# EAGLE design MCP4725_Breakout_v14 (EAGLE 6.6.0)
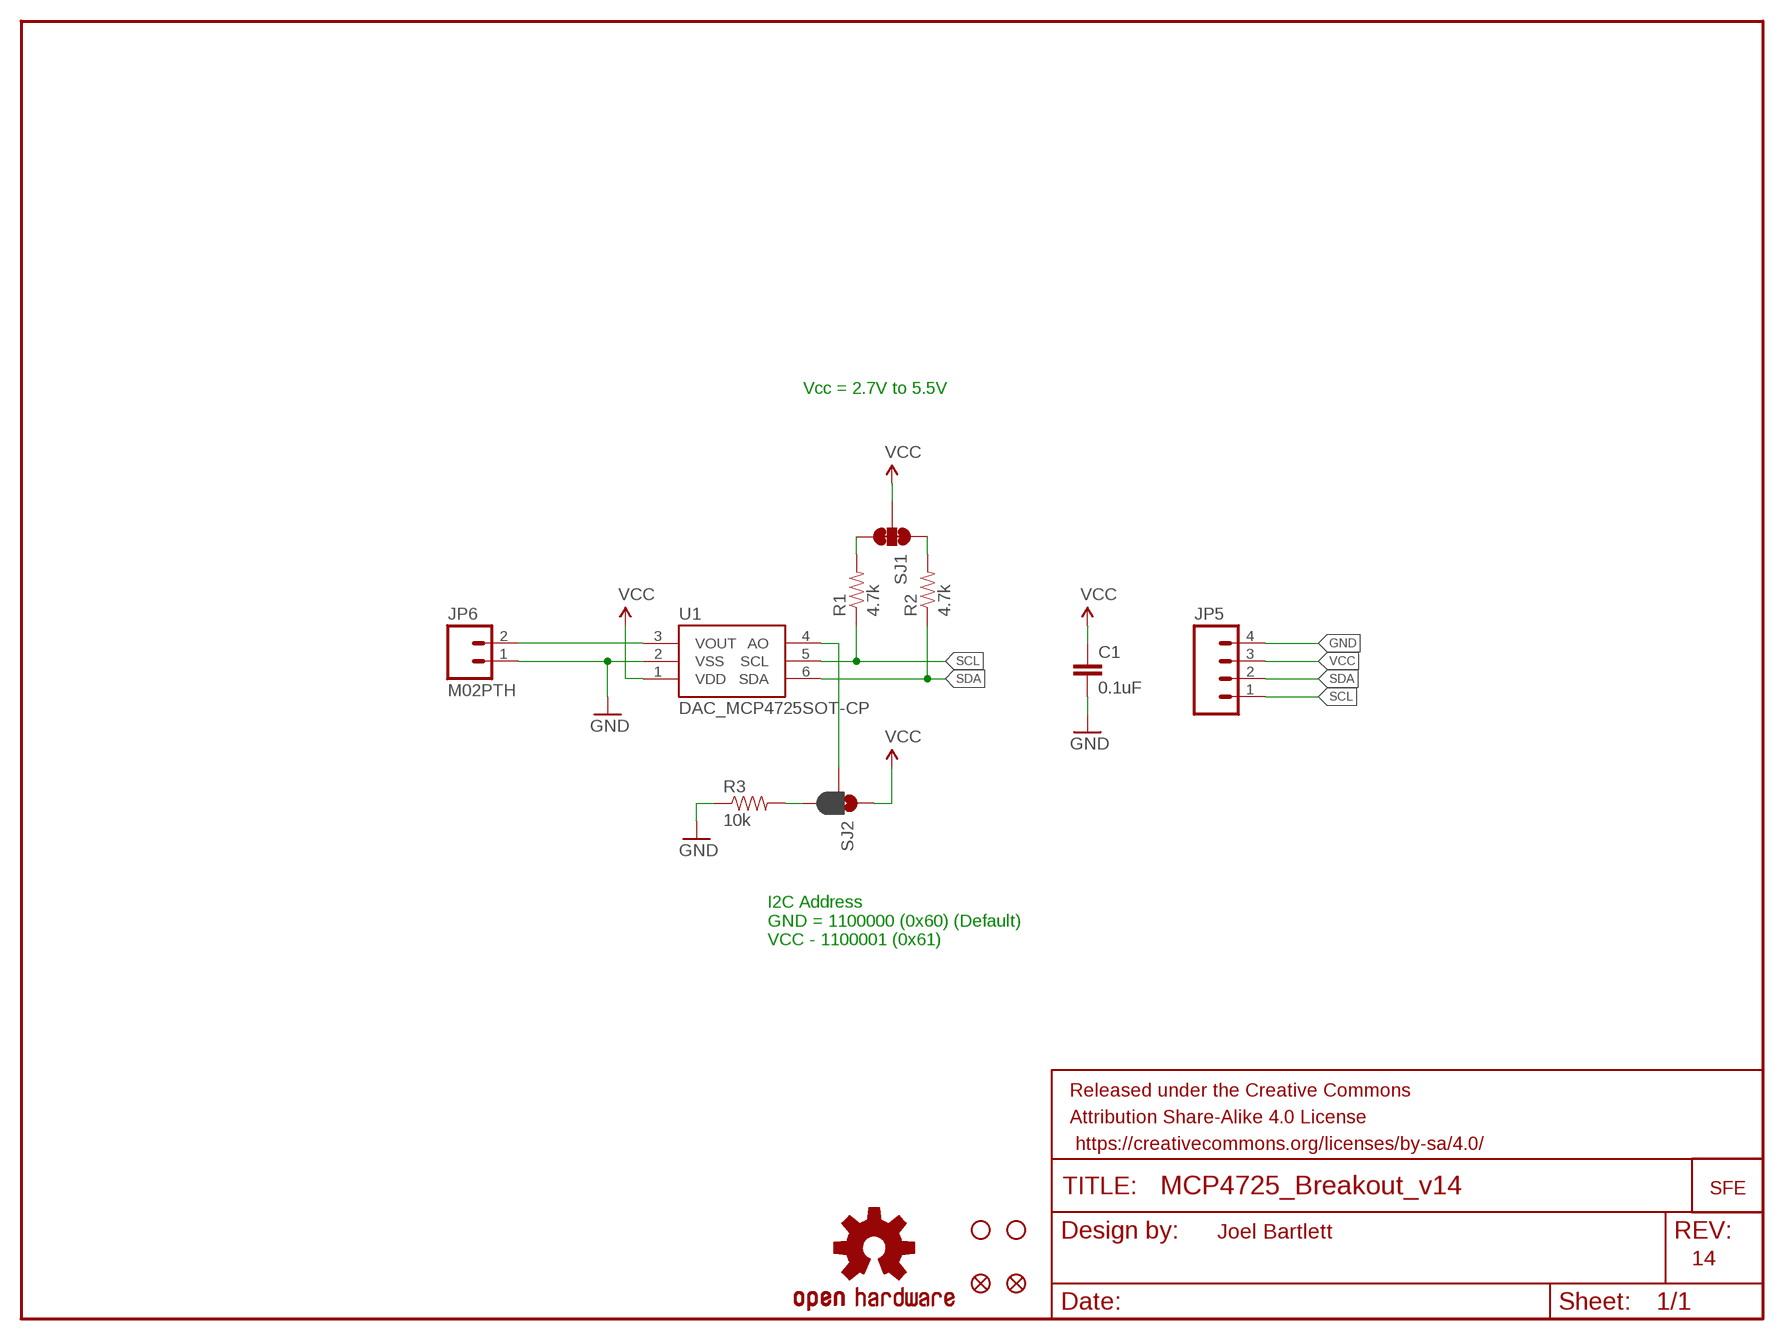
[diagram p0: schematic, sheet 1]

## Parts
C1  0.1uF  CAP0603-CAP  [0603-CAP]
FID1  FIDUCIAL1X2  [FIDUCIAL-1X2]
FID2  FIDUCIAL1X2  [FIDUCIAL-1X2]
FRAME2  FRAME-LETTER  [CREATIVE_COMMONS]
GND  LOGO-SFESK  [SFE-LOGO-FLAME]
JP5  M04PTH  [1X04]
JP6  M02PTH  [1X02]
LOGO1  OSHW-LOGOS  [OSHW-LOGO-S]
R1  4.7k  RESISTOR0603-RES  [0603-RES]
R2  4.7k  RESISTOR0603-RES  [0603-RES]
R3  10k  RESISTOR0603-RES  [0603-RES]
SJ1  JUMPER-PAD-3-NC_BY_TRACE  [PAD-JUMPER-3-3OF3_NC_BY_TRACE_YES_SILK_FULL_BOX]
SJ2  JUMPER-PAD-3-2OF3_NC_BY_PASTE  [PAD-JUMPER-3-2OF3_NC_BY_PASTE_YES_SILK_FULL_BOX]
STANDOFF1  STAND-OFF  [STAND-OFF]
STANDOFF2  STAND-OFF  [STAND-OFF]
U1  DAC_MCP4725SOT-CP  [SOT23-6-MCP4725]

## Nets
GND: C1.2 JP5.4 JP6.1 R3.1 U1.2(VSS)
N$1: R2.2 SJ1.1
N$2: R1.2 SJ1.3
N$3: SJ2.2 U1.4(AO)
N$4: R3.2 SJ2.3
SCL: JP5.1 R1.1 U1.5(SCL)
SDA: JP5.2 R2.1 U1.6(SDA)
VCC: C1.1 JP5.3 SJ1.2 SJ2.1 U1.1(VDD)
VOUT: JP6.2 U1.3(VOUT)

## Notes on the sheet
- Vcc = 2.7V to 5.5V
- I2C Address
  GND = 1100000 (0x60) (Default)
  VCC - 1100001 (0x61)
- Joel Bartlett
- 14

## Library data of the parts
C1 = SparkFun:CAP: Capacitor
FID1 FID2 = SparkFun-Aesthetics:FIDUCIAL: Fiducial Alignment Points
FRAME2 = SparkFun-Aesthetics:FRAME-LETTER: Schematic Frame
GND = SparkFun:LOGO-SFE: Spark Fun Electronics PCB Logo
JP5 = SparkFun-Connectors:M04: Header 4 Standard 4-pin 0.1" header. Use with straight break away headers (SKU : PRT-00116), right angle break away headers (PRT-00553), swiss pins (PRT-00743), machine pins (PRT-00117), and female headers (PRT-00115). Molex polarized connector foot print use with SKU : PRT-08231 with associated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
JP6 = SparkFun-Connectors:M02: Standard 2-pin 0.1" header. Use with
LOGO1 = SparkFun-Aesthetics:OSHW-LOGO: Open Source Hardware Logo This logo indicates the piece of hardware it is found on incorporates a OSHW license and/or adheres to the definition of open source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
R1-R3 = SparkFun:RESISTOR: Resistor
SJ1 = SparkFun-Passives:JUMPER-PAD-3-NC_BY_TRACE
SJ2 = SparkFun-Passives:JUMPER-PAD-3-2OF3_NC_BY_PASTE
STANDOFF1 STANDOFF2 = SparkFun-Electromechanical:STAND-OFF: #4 Stand Off
U1 = SparkFun-AnalogIC:DAC_MCP4725: Microchip 12-bit I2C DAC, SOT23-6

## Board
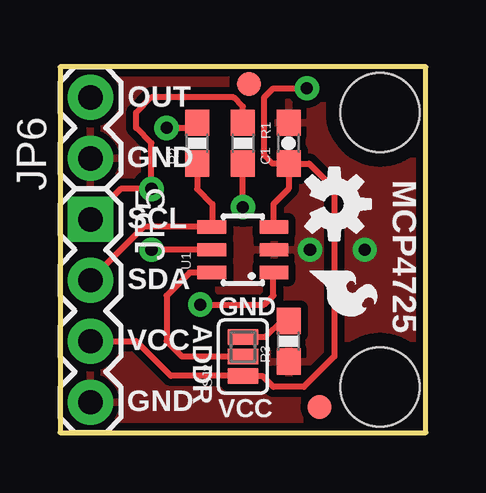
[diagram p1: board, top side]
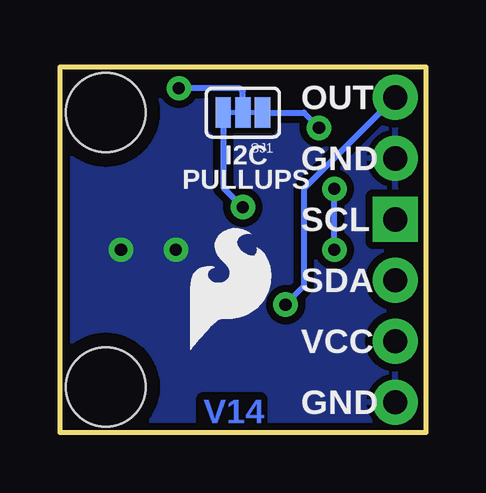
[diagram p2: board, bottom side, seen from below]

Size 15.24 x 15.24 mm. Coordinates in mm from the lower left corner, seen from the top.
Outline: 0,0 15.24,0 15.24,15.24 0,15.24 0,0
Copper layers (1*16): Top 0.035mm / dielectric 1.5mm / Bottom 0.035mm
Design rules "SparkFun-2-layer": minimum track width 7mil, minimum drill 15mil, track to track 8mil, track to pad 8mil, pad to pad 8mil, via to via 8mil, smd to smd 8mil, copper to edge 8mil, drill to drill 8mil, minimum pad ring 12mil, minimum via ring 10mil, stop-mask expansion 4mil, vias tented up to drill 20mil, thermal gap 10mil

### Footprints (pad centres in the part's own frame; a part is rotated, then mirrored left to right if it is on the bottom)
0603-CAP = smd 1.1 x 1: 1 -0.85,0; 2 0.85,0
FIDUCIAL-1X2 = smd 1 x 1: 1 0,0
1X04 = drill 1.016 pad 1.88 square: 1 0,0 | drill 1.016 pad 1.88: 2 2.54,0; 3 5.08,0; 4 7.62,0
1X02 = drill 1.016 pad 1.88: 1 0,0; 2 2.54,0
0603-RES = smd 1.1 x 1: 1 -0.85,0; 2 0.85,0
PAD-JUMPER-3-3OF3_NC_BY_TRACE_YES_SILK_FULL_BOX = smd 0.635 x 1.27: 1 -0.813,0; 2 0,0; 3 0.813,0
PAD-JUMPER-3-2OF3_NC_BY_PASTE_YES_SILK_FULL_BOX = smd 0.635 x 1.27: 1 -0.813,0; 2 0,0; 3 0.813,0
STAND-OFF = hole 3.302: 0,0
SOT23-6-MCP4725 = smd 0.55 x 1.2: 1 0.95,-1.3; 2 0,-1.3; 3 -0.95,-1.3; 4 -0.95,1.3; 5 0,1.3; 6 0.95,1.3

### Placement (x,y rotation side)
C1  9.53,12.06 90 top
FID1  10.82,1.07 0 top
FID2  7.87,14.53 0 top
FRAME2  not placed on the board
GND  10.41,6.73 270 top
JP5  1.27,8.89 270 top
JP6  1.27,11.43 90 top
LOGO1  11.43,9.53 270 top
R1  7.62,12.06 270 top
R2  5.71,12.06 90 top
R3  9.53,3.81 90 top
SJ1  7.62,13.34 180 bottom
SJ2  7.62,3.17 90 top
STANDOFF1  13.34,13.34 0 top
STANDOFF2  13.34,1.91 0 top
U1  7.62,7.62 90 top
U$3  [SFE_LOGO_FLAME_.2]  10.16,3.17 0 bottom

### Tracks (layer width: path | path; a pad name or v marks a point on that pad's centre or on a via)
GND  (via drill 0.51)
  other vias: 12.7,7.62 10.41,7.62
  pour Bottom (isolate 0.305): 0,15.24 0,0 15.24,0 15.24,15.24
  pour Top (isolate 0.305): 0,15.24 0,0 15.24,0 15.24,15.24
N$1  (via drill 0.51)
  Top 0.254: v4.45,12.7 5.5,12.7 R2.2
  Bottom 0.254: v4.45,12.7 5.08,13.34 SJ1.1
N$2  (via drill 0.51)
  Top 0.254: v7.62,9.4 R1.2
  Bottom 0.254: v7.62,9.4 8.43,10.21 SJ1.3
N$3
  Top 0.254: U1.4 5.4,6.67 4.45,5.71 4.45,3.81 5.08,3.17 SJ2.2
N$4
  Top 0.254: SJ2.3 8.56,3.99 9.23,4.66 R3.2
SCL  (via drill 0.51)
  Top 0.254: U1.5 v3.81,7.62 | JP5.1 2.54,10.16 v3.81,10.16 3.81,12.06 3.17,12.7 3.17,13.34 3.81,13.97 7.24,13.97 7.62,13.59 R1.1
  Bottom 0.254: v3.81,7.62 v3.81,10.16
SDA
  Top 0.254: JP5.2 3.49,8.57 U1.6 6.35,8.6 6.35,9.53 5.71,10.16 R2.1
VCC  (via drill 0.51)
  Top 0.254: JP5.3 3.17,3.81 4.62,2.36 SJ2.1 8.43,2.36 8.89,1.91 10.16,1.91 11.43,3.17 11.43,10.16 10.38,11.21 C1.1 | C1.1 8.85,11.21 8.51,11.56 8.51,13.97 8.89,14.35 v10.29,14.35 | C1.1 9.53,10.16 8.89,9.53 8.89,8.6 U1.1
  Bottom 0.254: SJ1.2 7.62,14.22 7.75,14.35 v10.29,14.35
VOUT  (via drill 0.51)
  Top 0.254: v5.84,5.33 8.51,5.33 8.89,5.71 8.89,6.64 U1.3
  Bottom 0.254: v5.84,5.33 5.08,6.1 5.08,10.16 JP6.2

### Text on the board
Bottom: V14
tPlace: OUT | GND | MCP4725 | SCL | SDA | ADDR | GND | VCC | GND | VCC
bPlace: OUT | GND | I2C | PULLUPS | SCL | SDA | VCC | GND
tDocu: Joel Bartlett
